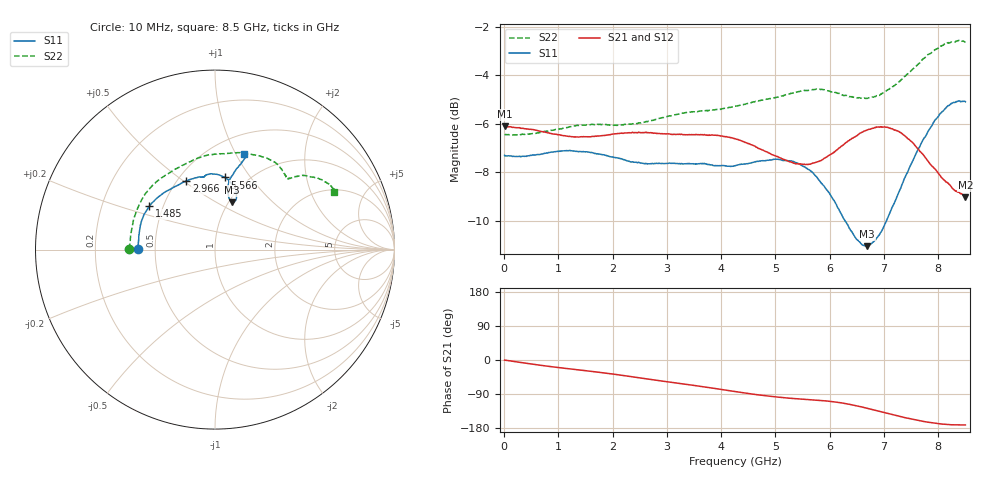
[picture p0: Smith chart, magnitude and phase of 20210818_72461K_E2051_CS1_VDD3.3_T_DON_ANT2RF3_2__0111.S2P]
!Agilent Technologies,E5071C,MY46417908,A.11.23
!Date: Wed Aug 18 14:31:07 2021
!Data & Calibration Information:
!Freq	S11:SOLT2(ON)	S21:SOLT2(ON)	S12:SOLT2(ON)	S22:SOLT2(ON)
!PortZ  Port1:50+j0  Port2:50+j0
!Above PortZ is port z conversion or system Z0 setting when saving the data.
!When reading, reference impedance value at option line is always used.
# Hz S dB R 50
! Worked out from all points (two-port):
!   1601 points, 10 MHz to 8.5 GHz, reference 50 ohm
!   highest |S21| = -6.11 dB at 10 MHz (marker M1); lowest = -9.0 dB at 8.5 GHz (marker M2)
!   |S21| within 3 dB of the highest: start of sweep to end of sweep
!   lowest |S11| = -11.1 dB at 6.691 GHz (marker M3), VSWR 1.78, Z = 52 + j29.7 ohm
!   |S11| at or under -10 dB: 6.279 GHz to 7.047 GHz (768.6 MHz wide, 11.5 % of centre)
!   |S22| runs from -6.5 to -2.6 dB; largest |S21 - S12| = 0.0027
!   S11 on the Smith chart (normalised r, x): 10 MHz: 0.40, +0.00; 1.485 GHz: 0.42, +0.25; 2.966 GHz: 0.55, +0.51; 5.566 GHz: 0.79, +0.76; 8.5 GHz: 0.70, +1.08
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1e7  -7.31 179.6  -6.11 -0.4  -6.11 -0.3  -6.43 179.6
7.847125e8  -7.21 163.4  -6.37 -16.1  -6.37 -16.1  -6.31 159.0
1.426769e9  -7.16 148.1  -6.54 -27.0  -6.55 -27.0  -6.06 140.0
1.485138e9  -7.16 146.6  -6.54 -28.0  -6.55 -28.0  -6.07 138.1
2.190869e9  -7.48 129.6  -6.41 -40.9  -6.41 -40.9  -6.06 118.5
2.843538e9  -7.64 115.1  -6.41 -54.3  -6.41 -54.3  -5.80 103.7
2.965581e9  -7.65 112.8  -6.42 -56.7  -6.42 -56.7  -5.73 101.4
3.591719e9  -7.66 102.9  -6.46 -69.0  -6.45 -69.1  -5.49 90.4
4.255e9  -7.74 98.4  -6.63 -83.2  -6.62 -83.3  -5.29 81.0
5.008488e9  -7.48 93.4  -7.34 -97.3  -7.35 -97.3  -4.93 69.8
5.565644e9  -7.83 82.4  -7.69 -104.0  -7.70 -104.0  -4.64 59.2
5.671769e9  -7.99 80.0  -7.65 -105.0  -7.67 -105.0  -4.61 57.2
6.128106e9  -9.37 69.8  -7.09 -111.3  -7.10 -111.5  -4.73 49.8
6.457094e9  -10.64 67.5  -6.56 -119.7  -6.55 -119.8  -4.93 45.9
6.690569e9  -11.06 69.9  -6.27 -127.5  -6.25 -127.6  -4.96 44.3
6.913431e9  -10.60 74.6  -6.15 -135.4  -6.14 -135.4  -4.84 43.8
7.088538e9  -9.79 77.2  -6.17 -141.8  -6.18 -141.8  -4.59 43.0
7.3114e9  -8.65 78.4  -6.39 -149.6  -6.39 -149.6  -4.21 41.6
7.497119e9  -7.69 77.5  -6.73 -155.6  -6.73 -155.7  -3.83 39.9
7.86325e9  -6.15 73.6  -7.70 -165.2  -7.67 -165.4  -3.09 34.3
8.144481e9  -5.35 71.7  -8.41 -169.8  -8.38 -169.9  -2.70 29.9
8.5e9  -5.10 73.0  -9.04 -171.5  -8.98 -171.4  -2.65 25.9
